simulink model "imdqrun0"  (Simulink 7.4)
settings: Solver=ode45  StartTime=0  StopTime=8  MaxStep=1e-3  RelTol=1e-3
InitFcn:
  | imparamrun0
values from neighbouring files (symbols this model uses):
  Bm = 0.10    (= 0.1)    [IMabc2.m]    (also in imabcparam.m = 0.01; IMabcrun0.m = 0.01; IMabcrun1.m = 0.001; IMcur0.m = 1e-06)
  fr0 = [phidr phiqr]    [imdef0vec.m]    (also in imdef1vec.m; imdefrotflux.m = sqrt(phidr^2+phiqr^2); imdefSIvec1.m)
  fs0 = fs    [calc0.m]    (also in imdef0vec.m = [phids phiqs]; imdef1vec.m = [phids phiqs]; imdefrotflux.m = [fs0d fs0q]; imdefSIvec1.m = [phids phiqs])
  J = 0.02    [imabcparam.m]    (also in IMabcrun0.m; IMabcrun1.m; imdefSIvec1.m = 0.03)
  Lm = eval(get(hLm,'String'))    [im3d.m]    (also in IMabc2.m = 4.5; imabcparam.m = 0.0847; IMabcrun0.m = 0.0847; IMabcrun1.m = 0.0847)
  Lrl = eval(get(hLr,'String'))    [im3d.m]    (also in IMabc2.m = 0.1; imabcparam.m = 0.0025; IMabcrun0.m = 0.0025; IMabcrun1.m = 0.0025)
  Lsl = eval(get(hLs,'String'))    [im3d.m]    (also in IMabc2.m = 0.1; imabcparam.m = 0.0025; IMabcrun0.m = 0.0025; IMabcrun1.m = 0.0025)
  nsync = 120*freq0/p    (= 1800)    [imabcparam.m]
  p = cos(beta-alpha)    [abcRwdg.m]    (also in alternator.m = 0:pi/20:2*pi; altwdgs.m = 0:pi/20:2*pi; brushlessdcB.m = 0:pi/100:2*pi; brushlessdcnew.m = 0:pi/100:2*pi)
  Rr = input('Rotor resistance)[default = 2] =')    [Actac.m]    (also in im1phase.m = 0.3; im3d.m = eval(get(hRr,'String')); IMabc2.m = 0.02; imabcparam.m = 0.408)
  Rs = eval(get(hRs,'String'))    [im3d.m]    (also in IMabc2.m = 0.01; imabcparam.m = 0.531; IMabcrun0.m = 0.531; IMabcrun1.m = 0.531)
  Vs = abs(Vas)    [calc0.m]    (also in Ccurverun.m = 1; IMabc2.m = 1; IMabcrun0.m = Vll*sqrt(2/3); IMabcrun1.m = Vll*sqrt(2/3))
  wk = ws    (= 1)    [imdef0vec.m]    (also in imdef1vec.m; imdef2vec.m; imdefrotflux.m; imdefSIvec1.m)
  wmec0 = n0*wo*2/p    (= 179.070781255)    [imdefSIvec1.m]
  wo = 2*pi*freq0    [calc0.m]    (also in IMabc2.m = 376.991118431; imabcparam.m = 376.991118431; IMabcrun0.m = 376.991118431; IMabcrun1.m = 376.991118431)
undefined symbols (not defined in the file or in its folder): TL1, TL2

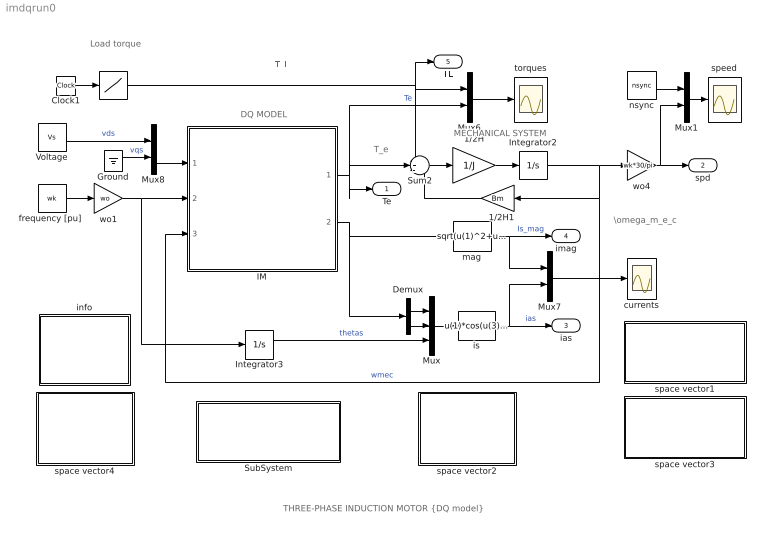
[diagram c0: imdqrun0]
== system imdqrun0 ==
  note: MECHANICAL SYSTEM
  note: DQ MODEL
  note: Load torque
  note: T_L
  note: \omega_m_e_c
  note: T_e
  note: THREE-PHASE INDUCTION MOTOR {DQ model}
  " " : Lookup  InputValues=[0 1.5 1.5 5 5 8]  Table="[TL1 TL1  TL2 TL2 TL1 TL1]"  OutDataType=sfix(16)  OutScaling=2^0
  1/2H : Gain  Gain=1/J  ParameterDataType=sfix(16)  ParameterScaling=2^0  OutDataType=sfix(16)  OutScaling=2^0
  1/2H1 : Gain  Gain=Bm  ParameterDataType=sfix(16)  ParameterScaling=2^0  OutDataType=sfix(16)  OutScaling=2^0
  Clock1 : Clock
  Demux : Demux  Outputs=2
  Ground : Ground
  IM : Subsystem
  Integrator2 : Integrator  InitialCondition=wmec0
  Integrator3 : Integrator
  Mux : Mux  Inputs=3
  Mux{1,6..8} (4 alike) : Mux  Inputs=2
  SubSystem : Subsystem
  Sum2 : Sum  Inputs=-+-  OutDataType=sfix(16)  OutScaling=2^0
  Voltage : Constant  Value=Vs  OutDataType=sfix(16)  OutScaling=2^0
  currents : Scope
  "frequency [pu] " : Constant  Value=wk  OutDataType=sfix(16)  OutScaling=2^0
  info : Subsystem
  is : Fcn  Expr=u(1)*cos(u(3))-u(2)*sin(u(3))
  mag : Fcn  Expr=sqrt(u(1)^2+u(2)^2)
  nsync : Constant  Value=nsync  OutDataType=sfix(16)  OutScaling=2^0
  space vector1 : Subsystem
  space vector2 : Subsystem
  space vector3 : Subsystem
  space vector4 : Subsystem
  speed : Scope
  torques : Scope
  wo1 : Gain  Gain=wo  ParameterDataType=sfix(16)  ParameterScaling=2^0  OutDataType=sfix(16)  OutScaling=2^0
  wo4 : Gain  Gain=wk*30/pi  ParameterDataType=sfix(16)  ParameterScaling=2^0  OutDataType=sfix(16)  OutScaling=2^0
  Te : Outport
  spd : Outport  Port=2
  ias : Outport  Port=3
  imag : Outport  Port=4
  TL : Outport  Port=5
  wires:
  Demux/1 -> Mux/1
  Demux/2 -> Mux/2
  Mux/1 -> is/1
  is/1 -> Mux7/2, ias/1  "ias"
  mag/1 -> Mux7/1, imag/1  "Is_mag"
  Sum2/1 -> 1/2H/1
  1/2H/1 -> Integrator2/1
  Mux6/1 -> torques/1
  Clock1/1 -> " "/1
  " "/1 -> Mux6/1, Sum2/1, TL/1
  Mux8/1 -> IM/1(vs)
  Voltage/1 -> Mux8/1  "vds"
  Ground/1 -> Mux8/2  "vqs"
  "frequency [pu] "/1 -> wo1/1
  wo1/1 -> Integrator3/1, IM/2(wk)
  Integrator3/1 -> Mux/3  "thetas"
  IM/1(Te) -> Sum2/2, Te/1, Mux6/2  "Te"
  IM/2(is) -> Demux/1, mag/1
  Integrator2/1 -> 1/2H1/1, IM/3(wmec), wo4/1  "wmec"
  Mux7/1 -> currents/1
  1/2H1/1 -> Sum2/3
  wo4/1 -> spd/1, Mux1/2
  Mux1/1 -> speed/1
  nsync/1 -> Mux1/1

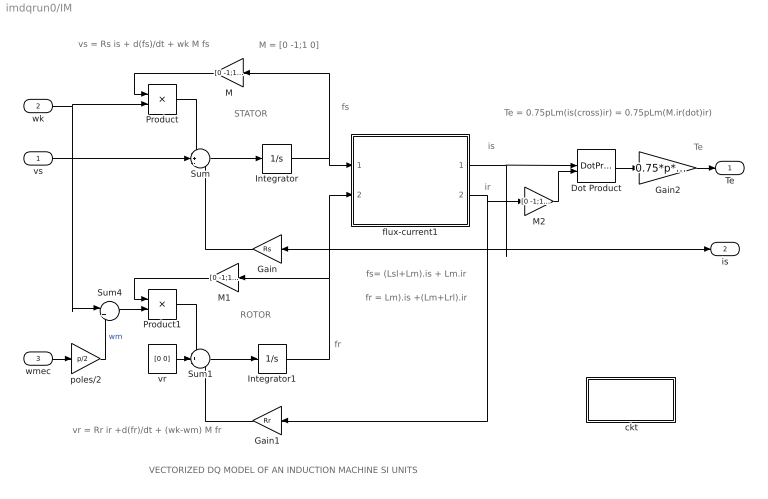
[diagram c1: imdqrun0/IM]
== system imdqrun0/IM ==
  note: ROTOR
  note: STATOR
  note: fs
  note: is
  note: Te
  note: VECTORIZED DQ MODEL OF AN INDUCTION MACHINE SI UNITS
  note: vs = Rs is + d(fs)/dt + wk M fs
  note: vr = Rr ir +d(fr)/dt + (wk-wm) M fr
  note: fs= (Lsl+Lm).is + Lm.ir
  note: fr = Lm).is +(Lm+Lrl).ir
  note: Te = 0.75pLm(is(cross)ir) = 0.75pLm(M.ir(dot)ir)
  note: M = [0 -1;1 0]
  note: ir
  note: fr
  vs : Inport  OutDataType=sfix(16)  OutScaling=2^0
  wk : Inport  Port=2  OutDataType=sfix(16)  OutScaling=2^0
  wmec : Inport  Port=3  OutDataType=sfix(16)  OutScaling=2^0
  " ckt" : Subsystem
  Dot Product : DotProduct  OutDataType=fixdt(1, 16)  OutScaling=2^-10
  Gain : Gain  Gain=Rs  ParameterDataType=sfix(16)  ParameterScaling=2^0  OutDataType=sfix(16)  OutScaling=2^0
  Gain1 : Gain  Gain=Rr  ParameterDataType=sfix(16)  ParameterScaling=2^0  OutDataType=sfix(16)  OutScaling=2^0
  Gain2 : Gain  Gain=0.75*p*Lm  ParameterDataType=sfix(16)  ParameterScaling=2^0  OutDataType=sfix(16)  OutScaling=2^0
  Integrator : Integrator  InitialCondition=fs0
  Integrator1 : Integrator  InitialCondition=fr0
  M : Gain  Gain=[0 -1;1 0]  Multiplication=Matrix(K*u)  ParameterDataType=sfix(16)  ParameterScaling=2^0  OutDataType=sfix(16)  OutScaling=2^0
  M1 : Gain  Gain=[0 -1;1 0]  Multiplication=Matrix(K*u)  ParameterDataType=sfix(16)  ParameterScaling=2^0  OutDataType=sfix(16)  OutScaling=2^0
  M2 : Gain  Gain=[0 -1;1 0]  Multiplication=Matrix(K*u)  ParameterDataType=sfix(16)  ParameterScaling=2^0  OutDataType=sfix(16)  OutScaling=2^0
  Product : Product  OutDataType=sfix(16)  OutScaling=2^0
  Product1 : Product  OutDataType=sfix(16)  OutScaling=2^0
  Sum : Sum  Inputs=-+-  OutDataType=sfix(16)  OutScaling=2^0
  Sum1 : Sum  Inputs=-+-  OutDataType=sfix(16)  OutScaling=2^0
  Sum4 : Sum  Inputs=|+-  OutDataType=sfix(16)  OutScaling=2^0
  flux-current1 : Subsystem
  poles/2 : Gain  Gain=p/2  ParameterDataType=sfix(16)  ParameterScaling=2^0  OutDataType=sfix(16)  OutScaling=2^0
  vr : Constant  Value=[0 0]  OutDataType=sfix(16)  OutScaling=2^0
  Te : Outport
  is : Outport  Port=2
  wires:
  Gain/1 -> Sum/3
  vr/1 -> Sum1/2
  Gain1/1 -> Sum1/3
  Integrator/1 -> M/1, flux-current1/1(fs)
  Integrator1/1 -> flux-current1/2(fr), M1/1
  Product1/1 -> Sum1/1
  M1/1 -> Product1/1
  Product/1 -> Sum/1
  M/1 -> Product/1
  Sum4/1 -> Product1/2
  vs/1 -> Sum/2
  wk/1 -> Product/2, Sum4/1
  Sum1/1 -> Integrator1/1
  Sum/1 -> Integrator/1
  flux-current1/1(is) -> Gain/1, is/1, Dot Product/1
  Dot Product/1 -> Gain2/1
  Gain2/1 -> Te/1
  wmec/1 -> poles/2/1
  poles/2/1 -> Sum4/2  "wm"
  M2/1 -> Dot Product/2
  flux-current1/2(ir) -> M2/1, Gain1/1

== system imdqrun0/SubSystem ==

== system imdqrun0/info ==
  note: The induction machine is modeled in vectorized form in conformity with the state vector formulation. This one-to-one correspondence can be seen by clicking both the INDUCTION MACHINE subsystem block and the MATHEMATICAL MODEL equation block. The synchronous reference frame is chosen here because the machine is operating under balanced three-phase sinusoidal excitation; the input voltage is thefore constant as indicated. The parameters describing the electromechanical system are expressed in SI units and may be modified by accessing a data file obtained by clicking the PARAMETERS block. In the present setup, the simulation portrays the dynamic response to a pulsed applied torque. The torque developed, the speed, and the stator current are observed on the scopes . The torque-speed dynamic characteristics can then be obtained after double clicking the PLOTS block. Press start button. To view the identical operation of this motor now modeled in abc phase variables, run the Matlab script file named > or double click block.
  note: Running of a Line-Fed Induction Motor Synchronous frame SI units

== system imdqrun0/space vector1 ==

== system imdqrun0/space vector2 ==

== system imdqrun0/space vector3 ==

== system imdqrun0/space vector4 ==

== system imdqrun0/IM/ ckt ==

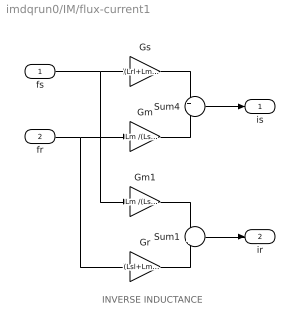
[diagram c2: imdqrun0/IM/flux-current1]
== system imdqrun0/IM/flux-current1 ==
  note: INVERSE INDUCTANCE
  fs : Inport  OutDataType=sfix(16)  OutScaling=2^0
  fr : Inport  Port=2  OutDataType=sfix(16)  OutScaling=2^0
  Gm : Gain  Gain=Lm /(Lsl*Lrl+Lsl*Lm+Lrl*Lm)  ParameterDataType=sfix(16)  ParameterScaling=2^0  OutDataType=sfix(16)  OutScaling=2^0
  Gm1 : Gain  Gain=Lm /(Lsl*Lrl+Lsl*Lm+Lrl*Lm)  ParameterDataType=sfix(16)  ParameterScaling=2^0  OutDataType=sfix(16)  OutScaling=2^0
  Gr : Gain  Gain=(Lsl+Lm )/(Lsl*Lrl+Lsl*Lm+Lrl*Lm)  ParameterDataType=sfix(16)  ParameterScaling=2^0  OutDataType=sfix(16)  OutScaling=2^0
  Gs : Gain  Gain=(Lrl+Lm) /(Lsl*Lrl+Lsl*Lm+Lrl*Lm)  ParameterDataType=sfix(16)  ParameterScaling=2^0  OutDataType=sfix(16)  OutScaling=2^0
  Sum1 : Sum  Inputs=-+  OutDataType=sfix(16)  OutScaling=2^0
  Sum4 : Sum  Inputs=+-  OutDataType=sfix(16)  OutScaling=2^0
  is : Outport
  ir : Outport  Port=2
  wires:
  fs/1 -> Gs/1, Gm1/1
  Gs/1 -> Sum4/1
  fr/1 -> Gm/1, Gr/1
  Gm/1 -> Sum4/2
  Sum4/1 -> is/1
  Gm1/1 -> Sum1/1
  Gr/1 -> Sum1/2
  Sum1/1 -> ir/1
